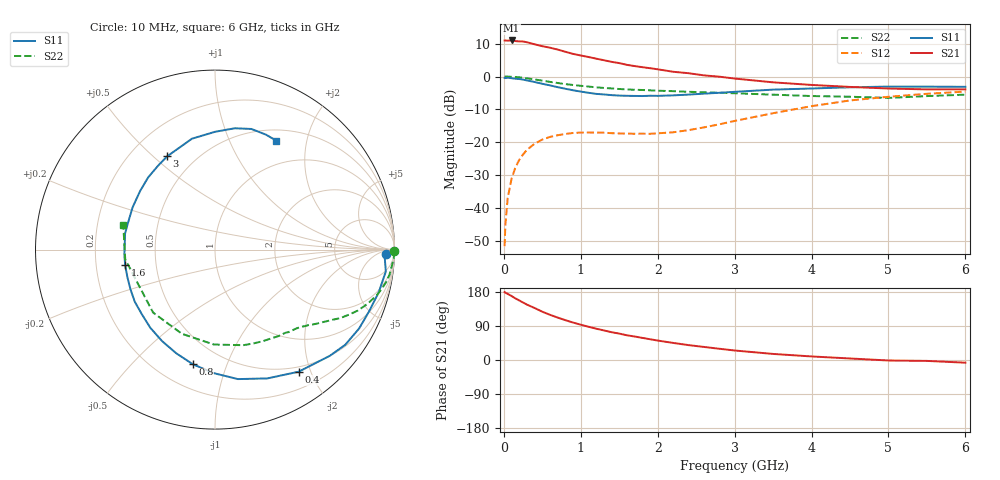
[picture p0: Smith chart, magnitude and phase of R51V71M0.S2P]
! SIEMENS Small Signal Semiconductors
! BFR183
! Si NPN RF Bipolar Junction Transistor in SOT23
! VCE = 1.75 V  IC = 1 mA
! Common Emitter S-Parameters:  May  1996
# GHz  S  MA  R  50
!  f  S11  S21  S12  S22
! GHz  MAG  ANG  MAG  ANG  MAG  ANG  MAG  ANG
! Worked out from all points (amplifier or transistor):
!   36 points, 10 MHz to 6 GHz, reference 50 ohm
!   highest |S21| = 11.0 dB at 100 MHz (marker M1)
!   |S21| within 3 dB of that: start of sweep to 732.7 MHz
!   unconditionally stable (mu >= 1): 1.623 GHz to 2.997 GHz
!   at 250 MHz: K = 0.16, MSG = 17.2 dB, |S12| = -23.7 dB
!   at 1.4 GHz: K = 0.86, MSG = 10.9 dB, |S12| = -17.3 dB
!   at 6 GHz: K = 0.97, MSG = 0.3 dB, |S12| = -4.6 dB
!   S11 on the Smith chart (normalised r, x): 10 MHz: 31, -18; 400 MHz: 0.43, -1.82; 800 MHz: 0.35, -0.76; 1.6 GHz: 0.33, -0.08; 3 GHz: 0.35, +0.55; 6 GHz: 0.64, +1.51
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0.01  0.9521 -1.6  3.534 179.2  0.0026 91.1  0.9986 -0.6
0.02  0.947 -2.8  3.539 177.6  0.0055 85.1  0.9981 -1.1
0.05  0.9595 -7.3  3.517 174.4  0.014 84.5  0.9969 -2.8
0.1  0.9424 -14.7  3.542 168.9  0.0276 81.4  0.989 -5.4
0.15  0.925 -21.8  3.466 162.6  0.0411 76.6  0.9819 -8.3
0.25  0.8987 -36.2  3.418 151.6  0.065 68.3  0.9548 -13.2
0.3  0.8713 -42.8  3.326 146.2  0.0763 65.1  0.938 -15.6
0.4  0.8246 -55.6  3.094 137.2  0.0946 58.2  0.9027 -19.5
0.5  0.7746 -67.9  2.896 127.4  0.1094 51.7  0.8654 -23.1
0.6  0.7326 -80.0  2.747 119.3  0.1202 46.6  0.8283 -26.0
0.7  0.688 -90.7  2.573 111.9  0.1275 42.0  0.7963 -28.6
0.8  0.6502 -101.0  2.378 105.1  0.1333 38.2  0.7648 -30.7
0.9  0.617 -110.4  2.211 98.8  0.138 35.4  0.7427 -32.4
1.1  0.5651 -129.7  1.982 87.8  0.1402 31.1  0.7023 -35.9
1.4  0.5204 -154.7  1.672 73.4  0.1369 28.7  0.6579 -40.4
1.6  0.5079 -170.1  1.505 65.2  0.1349 30.0  0.6356 -43.3
2.2  0.5158 152.9  1.181 45.1  0.1412 42.3  0.5981 -53.6
3  0.584 117.2  0.931 25.1  0.2104 54.8  0.5555 -73.5
3.5  0.6312 101.7  0.815 16.0  0.2761 53.4  0.529 -90.6
4.5  0.685 80.7  0.694 4.0  0.4318 40.1  0.492 -134.5
5.5  0.7005 66.1  0.636 -2.4  0.5452 23.1  0.5031 -173.9
6  0.6965 60.6  0.637 -7.1  0.5888 13.2  0.529 165.0
